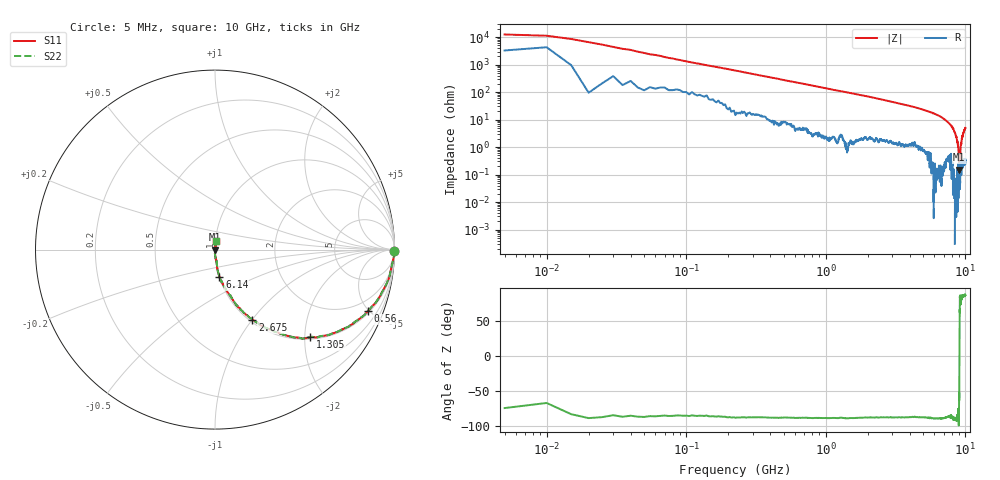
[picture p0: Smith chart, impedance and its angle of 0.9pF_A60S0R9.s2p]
! Amotech Co.,Ltd.
! http://www.amotech.co.kr/
! Part Number: A60S0R9
! These Parameters are Measured in Series Mode Connection
! Operation Temp=25[degC], DC Bias Voltage=0[V]
! Freq. Start=5[MHz] Stop=10[GHz], 2000[Steps]
! Date: Monday, July 13, 2020, 01:48:11
# GHZ S RI R 50.000000
!Freq.(Hz) S11(Real) S11(Imag) S21(Real) S21(Imag) S12(Real) S12(Imag) S22(Real) S22(Imag)
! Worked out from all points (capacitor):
!   2000 points, 5 MHz to 10 GHz, reference 50 ohm
!   read as one part in series: C = 1.21 pF near 55 MHz
!   lowest |Z| = 151 mohm at 9.05 GHz (marker M1)
!   series resonance near 9.064 GHz, so ESL is about 260 pH
!   S11 on the Smith chart (normalised r, x): 5 MHz: open; 560 MHz: 1.12, -4.91; 1.305 GHz: 1.05, -2.13; 2.675 GHz: 1.03, -1.00; 6.14 GHz: 1.00, -0.31; 10 GHz: 1.01, +0.10
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0.005  0.9979 -0.00769  0.00215 0.00769  0.00215 0.00769  0.9979 -0.00769
0.085  0.9908 -0.0634  0.00924 0.0634  0.00924 0.0634  0.9908 -0.0634
0.16  0.9798 -0.1156  0.0202 0.1156  0.0202 0.1156  0.9798 -0.1156
0.32  0.9417 -0.2177  0.0583 0.2177  0.0583 0.2177  0.9417 -0.2177
0.56  0.8519 -0.3433  0.1481 0.3433  0.1481 0.3433  0.8519 -0.3433
1.305  0.5306 -0.4874  0.4694 0.4874  0.4694 0.4874  0.5306 -0.4874
1.675  0.409 -0.4814  0.591 0.4814  0.591 0.4814  0.409 -0.4814
2.675  0.2088 -0.3907  0.7912 0.3907  0.7912 0.3907  0.2088 -0.3907
3.34  0.1393 -0.328  0.8607 0.328  0.8607 0.328  0.1393 -0.328
5.005  0.0558 -0.2126  0.9442 0.2126  0.9442 0.2126  0.0558 -0.2126
6.14  0.0244 -0.1521  0.9756 0.1521  0.9756 0.1521  0.0244 -0.1521
6.67  0.017 -0.1247  0.983 0.1247  0.983 0.1247  0.017 -0.1247
7.855  0.00789 -0.0631  0.9921 0.0631  0.9921 0.0631  0.00789 -0.0631
8.335  0.000396 -0.036  0.9996 0.036  0.9996 0.036  0.000396 -0.036
8.615  0.000947 -0.023  0.9991 0.023  0.9991 0.023  0.000947 -0.023
8.805  0.000475 -0.014  0.9995 0.014  0.9995 0.014  0.000475 -0.014
8.92  0.00139 -0.00819  0.9986 0.00819  0.9986 0.00819  0.00139 -0.00819
9.05  0.00121 -0.000901  0.9988 0.000901  0.9988 0.000901  0.00121 -0.000901
9.095  0.0018 0.00245  0.9982 -0.00245  0.9982 -0.00245  0.0018 0.00245
9.275  0.00255 0.0116  0.9975 -0.0116  0.9975 -0.0116  0.00255 0.0116
9.455  0.00346 0.0206  0.9965 -0.0206  0.9965 -0.0206  0.00346 0.0206
10  0.0058 0.0503  0.9942 -0.0503  0.9942 -0.0503  0.0058 0.0503
